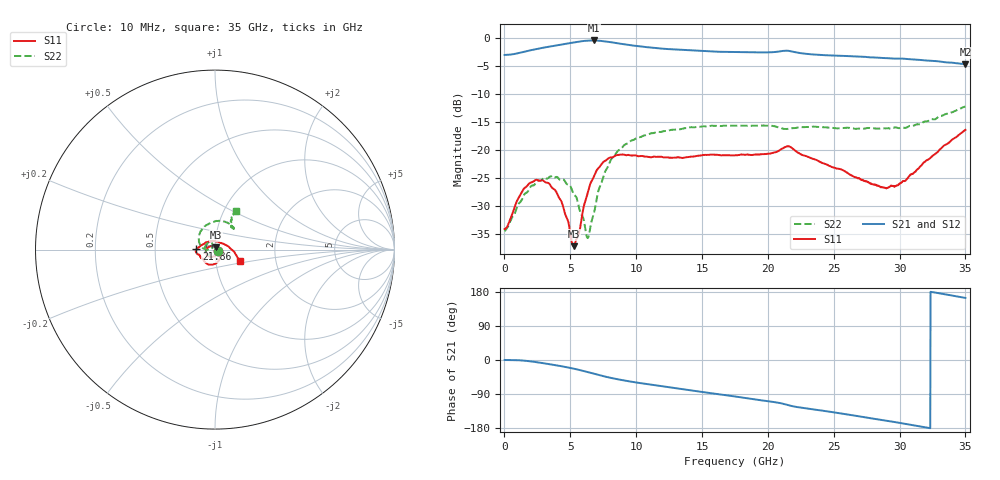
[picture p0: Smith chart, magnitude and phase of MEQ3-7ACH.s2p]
! MARKI MICROWAVE INC.
! Email:  support@markimicrowave.com  Phone:  408-778-4200
! Model Number:  MEQ3-7ACH  Date:  6/18
! Filename:		MEQ3-7ACH.S2P  Version: 1.0
! Description:  2-port S-parameter data for chip equalizer
! Features:		Low Insertion Loss, Excellent Return Loss
! Frequency Measured: 	10 MHz to 35 GHz
!S2P File: Measurements: S11, S12, S21, S22:
# Hz S  dB  R 50
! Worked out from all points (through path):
!   1601 points, 10 MHz to 35 GHz, reference 50 ohm
!   highest |S21| = -0.38 dB at 6.767 GHz (marker M1); lowest = -4.6 dB at 35 GHz (marker M2)
!   group delay of S21, straight-line fit = 15.8 ps
!   lowest |S11| = -37.2 dB at 5.258 GHz (marker M3), VSWR 1.03, Z = 50.3 + j1.35 ohm
!   |S11| at or under -10 dB: start of sweep to end of sweep
!   |S22| runs from -35.8 to -12.2 dB; largest |S21 - S12| = 0.0078
!   S11 on the Smith chart (normalised r, x): 10 MHz: 1.04, -0.02; 21.86 GHz: 0.81, +0.00; 35 GHz: 1.31, -0.17
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1e7  -34.16 -22.3  -2.98 0.1  -2.98 0.3  -34.59 -21.6
1.453338e9  -26.98 -113.3  -2.43 -1.6  -2.43 -1.6  -28.20 -118.8
2.28435e9  -25.49 -142.6  -1.98 -5.0  -1.98 -5.0  -26.20 -155.6
2.874806e9  -25.43 -161.7  -1.71 -8.0  -1.71 -8.0  -25.23 -177.4
3.443394e9  -26.17 -179.2  -1.47 -11.2  -1.47 -11.2  -24.76 163.9
4.230669e9  -28.82 155.7  -1.16 -15.9  -1.16 -15.9  -25.34 142.2
5.2585e9  -37.23 76.3  -0.74 -22.8  -0.74 -22.8  -27.94 117.4
5.586531e9  -35.41 13.6  -0.61 -25.4  -0.61 -25.4  -29.53 115.2
5.848956e9  -32.48 -10.7  -0.52 -27.6  -0.53 -27.5  -31.65 111.9
6.3082e9  -27.80 -42.4  -0.41 -31.7  -0.41 -31.7  -35.78 142.1
6.767444e9  -24.89 -62.8  -0.38 -35.9  -0.38 -35.9  -31.56 -179.1
7.270425e9  -22.86 -80.5  -0.45 -40.6  -0.44 -40.6  -26.44 -177.9
8.254519e9  -21.25 -105.9  -0.76 -48.5  -0.75 -48.5  -21.26 163.1
9.588512e9  -20.98 -126.4  -1.23 -57.0  -1.23 -57.0  -18.37 137.0
1.168791e10  -21.23 -139.0  -1.81 -68.0  -1.78 -68.0  -16.75 108.8
1.7505e10  -20.92 -155.2  -2.47 -96.3  -2.45 -96.4  -15.67 67.3
2.104774e10  -19.79 -166.3  -2.28 -114.6  -2.22 -115.0  -16.12 53.0
2.185688e10  -19.69 178.8  -2.38 -121.8  -2.38 -122.1  -16.09 54.4
2.334396e10  -21.51 167.1  -2.87 -129.7  -2.83 -129.7  -15.84 51.0
2.918291e10  -26.69 72.0  -3.57 -161.1  -3.53 -161.5  -16.10 51.5
3.047317e10  -25.44 38.1  -3.68 -168.8  -3.70 -168.9  -16.04 55.3
3.5e10  -16.39 -24.9  -4.62 163.9  -4.58 164.0  -12.21 61.8
